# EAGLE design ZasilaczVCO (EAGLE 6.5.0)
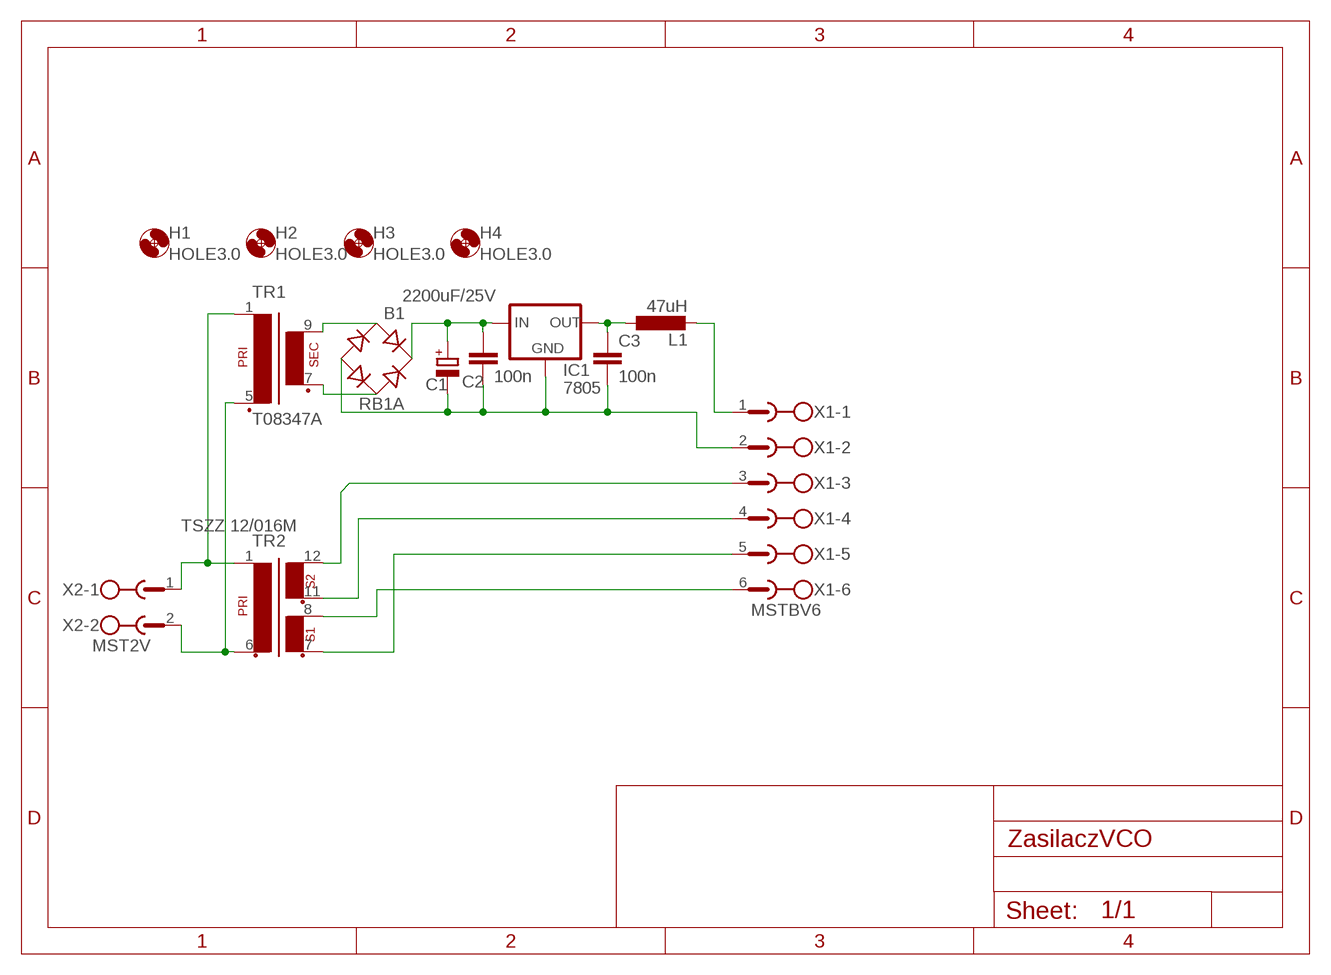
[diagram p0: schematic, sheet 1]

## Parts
B1  RB1A  RECTIFIER-RB1A  [RB1A]
C1  2200uF/25V  CPOL-EUE7.5-16  [E7,5-16]
C2  100n  C-EU025-024X044  [C025-024X044]
C3  100n  C-EU025-024X044  [C025-024X044]
H1  HOLE3.0  MOUNT-HOLE3.0  [3,0]
H2  HOLE3.0  MOUNT-HOLE3.0  [3,0]
H3  HOLE3.0  MOUNT-HOLE3.0  [3,0]
H4  HOLE3.0  MOUNT-HOLE3.0  [3,0]
IC1  7805  78XXS  [78XXS]
L1  47uH  L-EU2200-15.24  [2200-15.24]
TR1  T08347A  EI30-1  [EI30-1]
TR2  TSZZ 12/016M  EP07,5  [EP07,5]
X1  MSTBV6  [MSTBV6]
X2  MST2V  [MSTBV2]

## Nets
N$1: TR1.1 TR2.1 X2.1
N$2: TR1.5(P2) TR2.6 X2.2
N$3: B1.AC1 TR1.9(S4)
N$4: TR2.12 X1.3
N$5: L1.2 X1.1
N$6: TR2.11 X1.4
N$8: C3.1 IC1.OUT L1.1
N$9: TR2.8 X1.6
N$10: TR2.7 X1.5
N$14: B1.+ C1.+ C2.1 IC1.IN
N$15: B1.AC2 TR1.7(S3)
N$16: B1.- C1.- C2.2 C3.2 IC1.GND X1.2

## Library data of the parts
B1 = rectifier:RECTIFIER-: Rectifier
C1 = rcl:CPOL-EU: POLARIZED CAPACITOR, European symbol
C2 C3 = rcl:C-EU: CAPACITOR, European symbol
H1-H4 = holes (2):MOUNT-HOLE: MOUNTING HOLE with drill center marker
IC1 = v-reg:78XXS: VOLTAGE REGULATOR
L1 = rcl:L-EU: INDUCTOR, European symbol
TR1 = trafo:EI30-1: TRANSFORMER 1 primary winding, 1 secondary winding ERA
TR2 = trafo:EP07,5: TRANSFORMER 1 primary winding, 2 secondary windings BLOCK
X1 = con-phoenix-508:MSTBV6: PHOENIX; MPN: MSTBV 2,5/6-GF-5.08; OC_FARNELL: 1792796; OC_NEWARK: 69R9849
X2 = con-phoenix-508:MST2V: PHOENIX; OC_FARNELL: unknown; OC_NEWARK: unknown

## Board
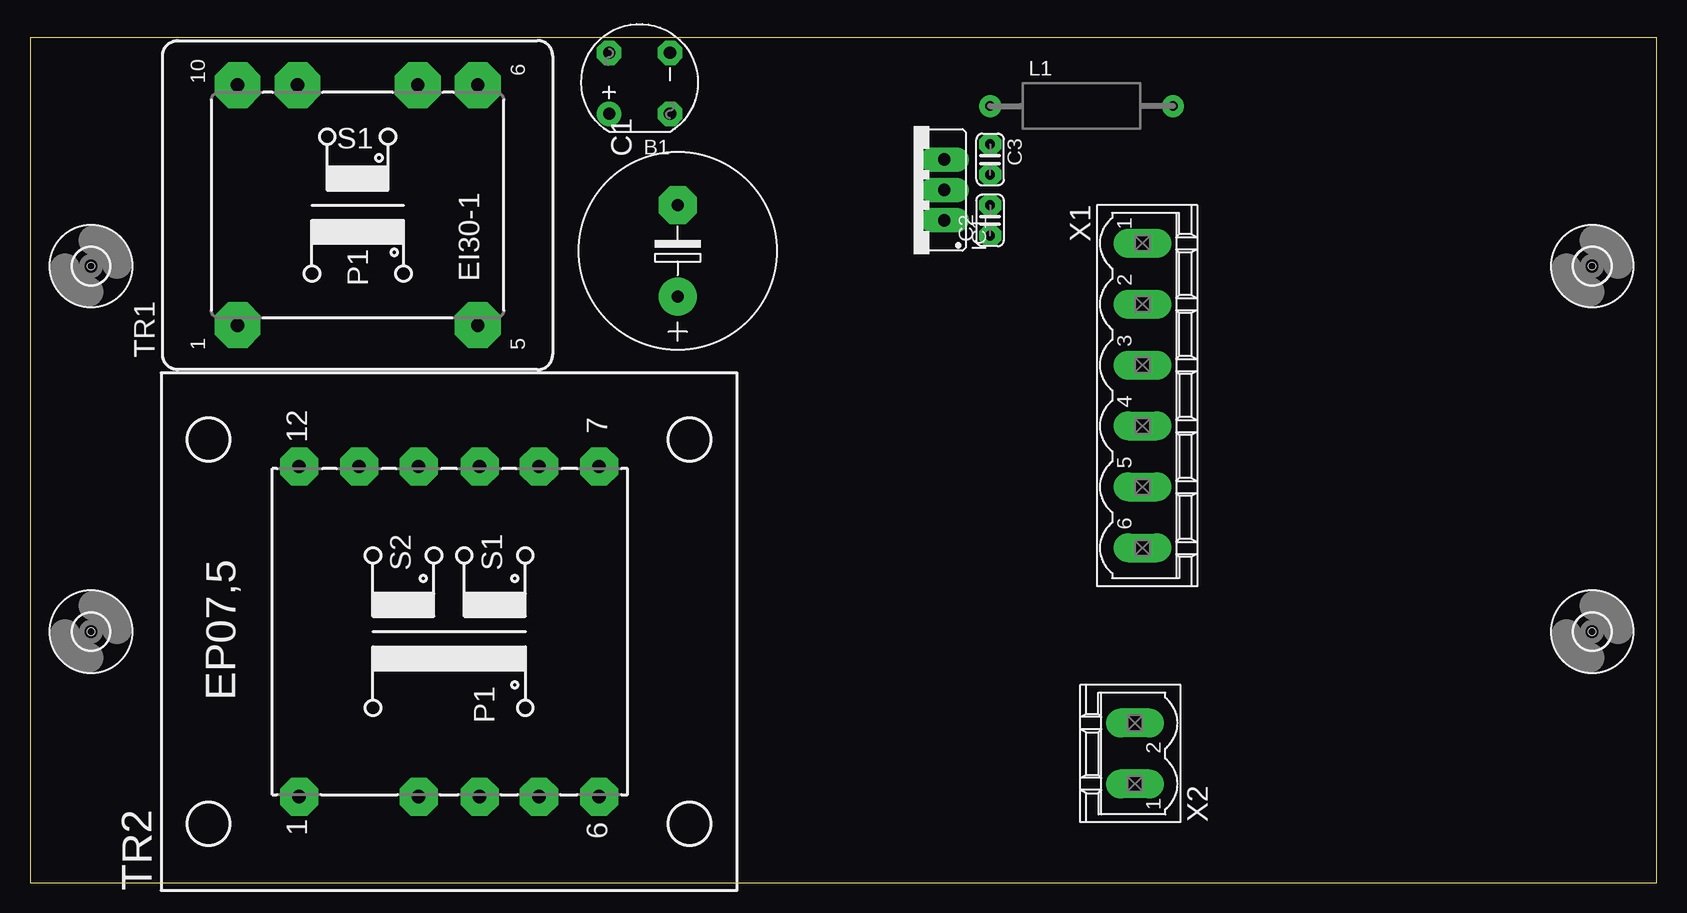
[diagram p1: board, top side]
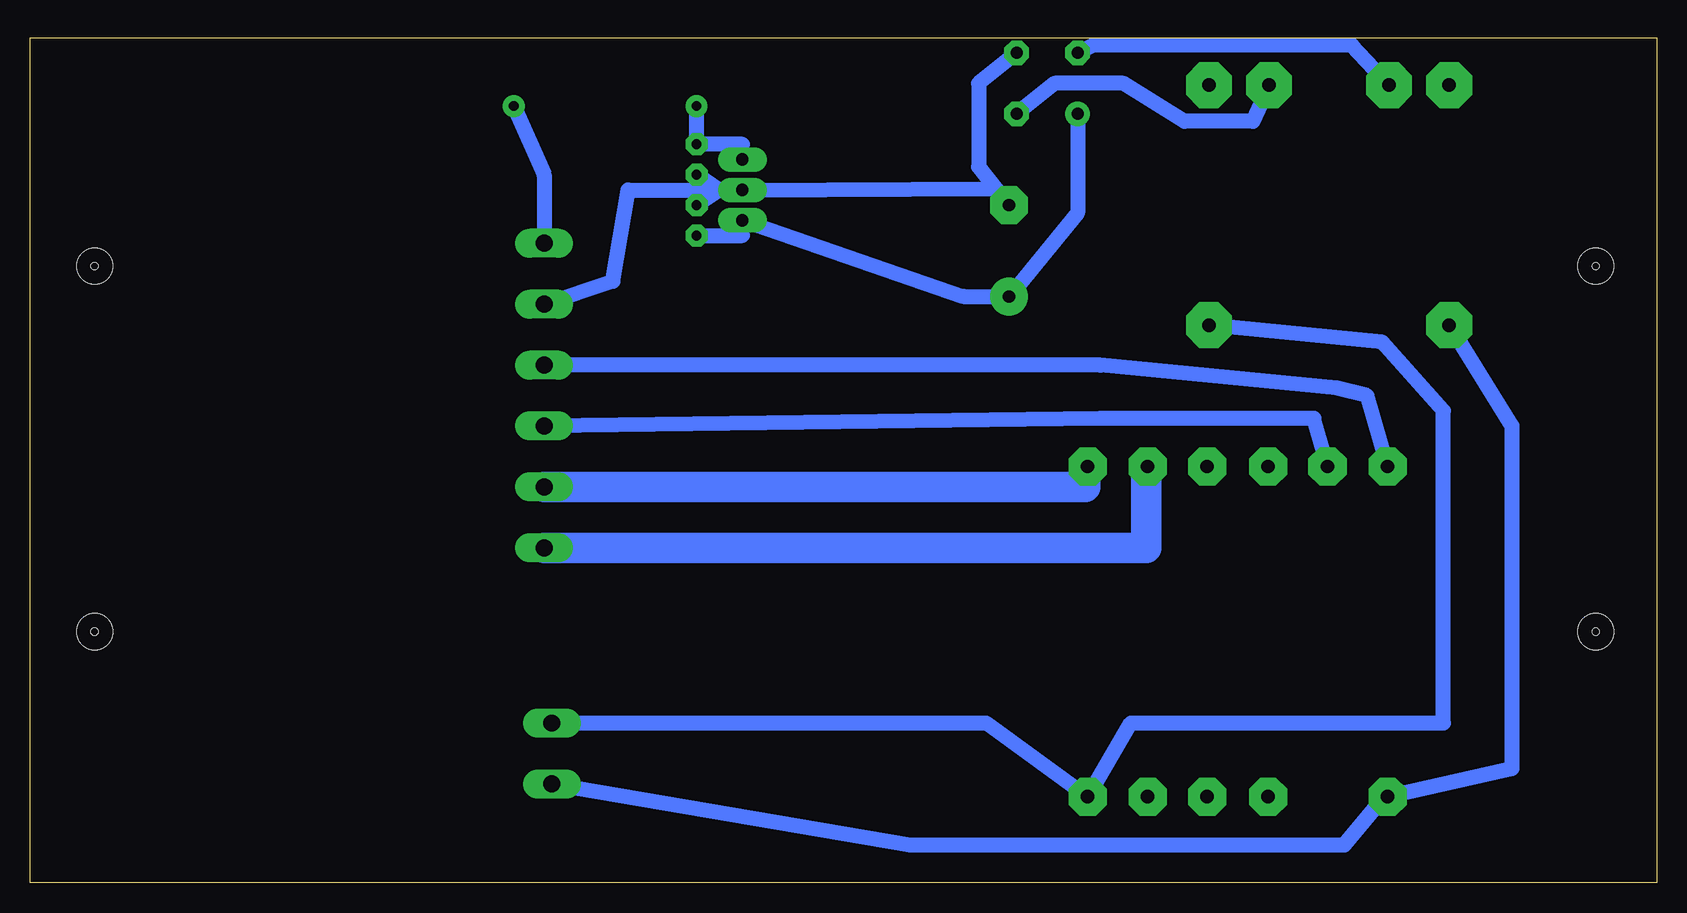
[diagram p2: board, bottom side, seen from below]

Size 135.56 x 70.47 mm. Coordinates in mm from the lower left corner, seen from the top.
Outline: 0,0 135.56,0 135.56,70.47 0,70.47 0,0
Copper layers (1*16): Top 0.035mm / dielectric 1.5mm / Bottom 0.035mm
Design rules "default *": minimum track width 50mil, minimum drill 24mil, track to track 8mil, track to pad 8mil, pad to pad 8mil, via to via 8mil, smd to smd 8mil, copper to edge 40mil, drill to drill 8mil, minimum pad ring 20mil, minimum via ring 8mil, stop-mask expansion 4mil, vias tented up to drill 0mil, thermal gap 10mil
Holes 0.6 mm at 5.08,20.95 5.08,51.44 130.18,20.95 130.18,51.44

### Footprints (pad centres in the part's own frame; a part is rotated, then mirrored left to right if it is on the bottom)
RB1A = drill 1.016: + -2.54,2.54 | drill 1.016 octagon: - 2.54,-2.54; AC1 2.54,2.54; AC2 -2.54,-2.54
E7,5-16 = drill 1.016 pad 3.15: + -3.81,0 | drill 1.016 pad 3.15 octagon: - 3.81,0
C025-024X044 = drill 0.813 octagon: 1 -1.27,0; 2 1.27,0
3,0 = hole 3: 0,0
78XXS = drill 1.016 long: GND 0,-2.54; IN -2.54,-2.54; OUT 2.54,-2.54
2200-15.24 = drill 0.8 pad 1.27: 1 -7.62,0; 2 7.62,0
EI30-1 = drill 1.118 pad 3.81 octagon: 1 -10.008,10.008; 5 -10.008,-10.008; 6 10.008,-10.008; 7 10.008,-5.004; 9 10.008,5.004; 10 10.008,10.008
EP07,5 = drill 1.118 pad 3.175 octagon: 1 -13.767,12.497; 3 -13.767,2.54; 4 -13.767,-2.54; 5 -13.767,-7.493; 6 -13.767,-12.497; 7 13.767,-12.497; 8 13.767,-7.493; 9 13.767,-2.54; 10 13.767,2.54; 11 13.767,7.493; 12 13.767,12.497
MSTBV6 = drill 1.397 long: 1 -12.7,0; 2 -7.62,0; 3 -2.54,0; 4 2.54,0; 5 7.62,0; 6 12.7,0
MSTBV2 = drill 1.397 long: 1 -2.54,0; 2 2.54,0

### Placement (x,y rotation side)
B1  50.8,66.67 90 top
C1  53.98,52.7 90 top
C2  80.01,55.24 90 top
C3  80.01,60.33 270 top
H1  MOUNT-HOLE3.0  [3,0]  130.18,51.44 0 top
H2  MOUNT-HOLE3.0  [3,0]  130.18,20.95 0 top
H3  MOUNT-HOLE3.0  [3,0]  5.08,51.44 0 top
H4  MOUNT-HOLE3.0  [3,0]  5.08,20.95 0 top
IC1  73.66,57.78 90 top
L1  87.63,64.77 0 top
TR1  [EI30-1]  27.3,56.52 90 top
TR2  34.92,20.95 90 top
X1  92.71,40.64 270 top
X2  92.08,10.79 90 top

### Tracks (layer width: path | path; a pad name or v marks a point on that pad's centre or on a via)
N$1
  Bottom 1.27: TR1.1 12.06,38.1 12.06,9.53 TR2.1 22.86,6.99 26.04,3.17 62.23,3.17 X2.1
N$2
  Bottom 1.27: X2.2 55.88,13.34 TR2.6 43.81,13.34 17.78,13.34 17.78,39.37 22.86,45.09 TR1.5
N$3
  Bottom 1.27: TR1.9 25.4,69.85 46.99,69.85 B1.AC1
N$4
  Bottom 1.27: TR2.12 24.13,40.64 26.67,41.27 46.35,43.18 X1.3
N$5
  Bottom 1.27: L1.2 92.71,59.05 X1.1
N$6
  Bottom 1.27: TR2.11 28.57,38.73 46.35,38.73 X1.4
N$8
  Bottom 1.27: IC1.OUT 76.2,61.59 C3.1 L1.1
N$9
  Bottom 1.27: TR2.8 42.55,34.92
  Bottom 2.54: X1.6 42.55,27.94 42.55,34.92
N$10
  Bottom 1.27: X1.5 48.26,33.02 TR2.7
  Bottom 2.54: X1.5 47.62,33.02 47.62,34.92
N$14
  Bottom 1.27: B1.+ 48.26,55.88 C1.+ 57.78,48.9 IC1.IN 76.2,53.98 C2.1
N$15
  Bottom 1.27: TR1.7 33.66,63.5 39.37,63.5 44.45,66.67 50.16,66.67 B1.AC2
N$16
  Bottom 1.27: B1.- 56.52,66.67 56.52,59.69 55.09,57.91 | 55.09,57.91 C1.- | C3.2 78.11,57.78 | 78.11,57.78 IC1.GND | C2.2 78.11,57.78 | IC1.GND 55.09,57.91 | X1.2 87,50.16 85.72,57.78 IC1.GND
